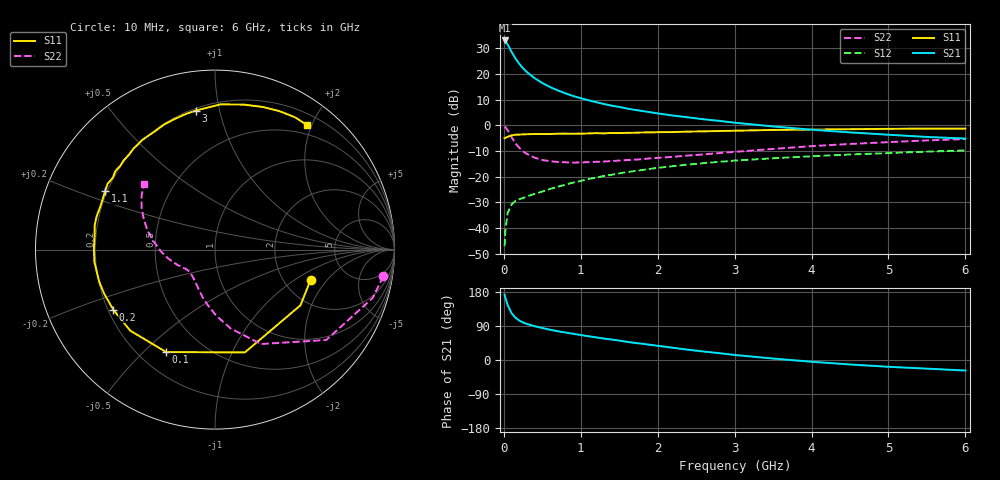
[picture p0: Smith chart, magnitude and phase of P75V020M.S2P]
! SIEMENS Small Signal Semiconductors
! BFP196
! Si NPN RF Bipolar Junction Transistor in SOT143
! VCE = 5 V  IC = 20 mA
! Common Emitter S-Parameters:  May  1996
# GHz  S  MA  R  50
!  f  S11  S21  S12  S22
! GHz  MAG  ANG  MAG  ANG  MAG  ANG  MAG  ANG
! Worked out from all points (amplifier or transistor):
!   36 points, 10 MHz to 6 GHz, reference 50 ohm
!   highest |S21| = 33.1 dB at 10 MHz (marker M1)
!   |S21| within 3 dB of that: start of sweep to 75.14 MHz
!   unconditionally stable (mu >= 1): 706 MHz to 3.46 GHz
!   at 250 MHz: K = 0.59, MSG = 25.2 dB, |S12| = -28.3 dB
!   at 1.4 GHz: K = 1.10, MAG = 11.5 dB, |S12| = -19.3 dB
!   at 6 GHz: K = 0.96, MSG = 2.3 dB, |S12| = -9.8 dB
!   S11 on the Smith chart (normalised r, x): 10 MHz: 2.80, -1.36; 100 MHz: 0.31, -0.59; 200 MHz: 0.22, -0.26; 1.1 GHz: 0.19, +0.24; 3 GHz: 0.21, +0.85; 6 GHz: 0.36, +1.93
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0.01  0.5589 -17.4  44.98 172.5  0.0044 82.9  0.9492 -9.0
0.02  0.5684 -33.1  43.05 164.0  0.009 77.9  0.9193 -17.0
0.05  0.5964 -73.8  37.49 144.8  0.0195 61.7  0.7985 -39.1
0.1  0.6325 -115.5  27.09 123.8  0.0287 46.9  0.5848 -64.1
0.15  0.6535 -136.3  20.1 111.8  0.0335 41.9  0.4476 -78.8
0.2  0.6581 -149.5  15.84 104.2  0.0361 40.9  0.3648 -89.4
0.25  0.6644 -158.1  12.87 98.9  0.0385 41.3  0.3092 -97.9
0.3  0.6694 -164.4  10.87 95.1  0.0408 42.3  0.277 -104.0
0.4  0.6752 -173.9  8.29 89.3  0.046 44.6  0.2333 -113.9
0.5  0.6749 179.5  6.656 84.4  0.0511 47.1  0.2105 -121.4
0.6  0.6751 173.7  5.565 80.0  0.0573 49.2  0.1991 -127.1
0.7  0.6838 168.5  4.792 75.9  0.0631 50.6  0.1929 -131.6
0.9  0.6824 160.2  3.728 69.2  0.0763 52.2  0.1874 -138.3
1.1  0.6932 152.1  3.075 62.7  0.0893 52.8  0.1912 -143.0
1.3  0.6959 144.8  2.602 56.7  0.1026 51.6  0.1965 -147.3
1.6  0.7114 135.6  2.119 48.0  0.1221 49.9  0.2098 -152.4
2.2  0.7375 117.9  1.545 32.2  0.1598 44.0  0.2427 -162.7
3  0.7822 97.8  1.123 13.3  0.2047 34.3  0.3032 -178.5
3.5  0.8098 87.8  0.948 3.8  0.2273 28.1  0.346 172.3
4.5  0.8385 71.3  0.726 -11.8  0.269 17.0  0.4317 156.8
5.5  0.8616 58.7  0.592 -22.8  0.3059 6.2  0.5063 143.9
6  0.8629 53.5  0.551 -27.8  0.3233 0.3  0.5392 137.6
